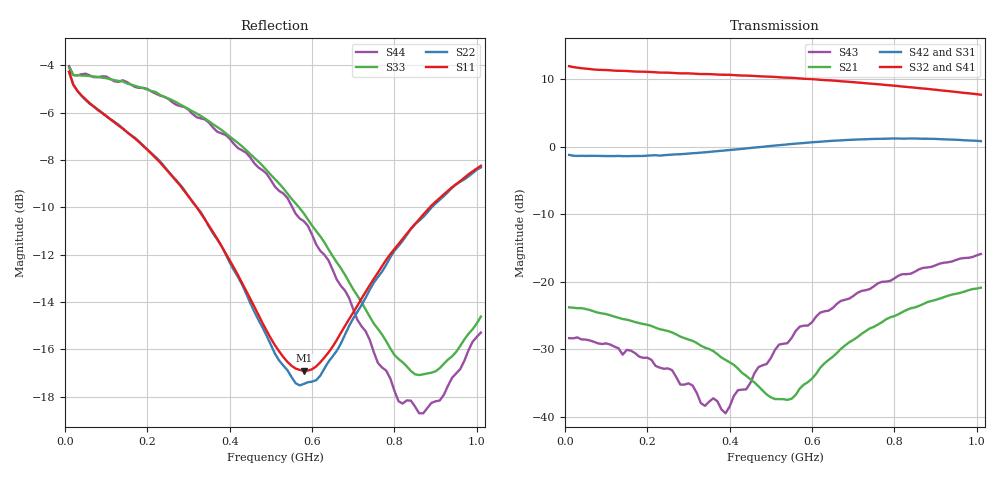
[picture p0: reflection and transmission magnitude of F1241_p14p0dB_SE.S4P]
! Integrated Device Technology
! Corporate Headquarters
! 6024 Silver Creek Valley Road
! San Jose, CA 95138  USA
! Phone:  1-408-284-8200
! Toll Free:  1-800-223-1366
! Webpage:  http://www.idt.com/
! Timing and RF Division
! 515 Groton Road, Suite 102
! Westford, MA 01886-6024
! Device:  F1241
! Description: Dual Intermediate Frequency Digital Variable Gain Amplifier
! Frequency:  10.0 -  500.00 MHz
! Package:  5x5 mm QFN Plastic Package: 32 pin
! Ports:  8 RF, 20 DC
!  Pin  1  = GA3  Pin 17  = RF OUT_B+
!  Pin  2  = GA4  Pin 18  = RF OUT_B-
!  Pin  3  = GA5  Pin 19  = STBY_B
!  Pin  4  = ISET_A  Pin 20  = Ground
!  Pin  5  = ISET_B  Pin 21  = Ground
!  Pin  6  = GB5  Pin 22  = STB_A
!  Pin  7  = GB4  Pin 23  = RF OUT_A-  = Port 4
!  Pin  8  = GB3  Pin 24  = RF OUT_A+  = Port 3
!  Pin  9  = GB2  Pin 25  = NO CONNECT
!  Pin 10  = GB1  Pin 26  = NO CONNECT
!  Pin 11  = RF IN_B+  Pin 27  = VCC
!  Pin 12  = RF IN_B-  Pin 28  = Ground
!  Pin 13  = Ground  Pin 29  = RF IN_A-  = Port 2
!  Pin 14  = VCC  Pin 30  = RF IN_A+  = Port 1
!  Pin 15  = NO CONNECT  Pin 31  = GA1
!  Pin 16  = NO CONNECT  Pin 32  = GA2
! State:  6
! Gain State:  14.0 dB
! Voltages:  Vcc = +5.00 Volts  Icc approximately 160.0 mA or 80 mA per channel.
! Data:  The device was measured on a custom evaluation board which has
!  individual transmission lines to the RF pins.  Data was collected
!  using a calibrated network analyzer.  The evaluation board was
!  de-embedded using a port reference technique.
!  The reference plane is the edge of the package pin.
!  Only Channel A was measured.
!  This data is in single-ended operation.  If your needs are balanced
!  or differential S-parameters then this file needs to be used a
!  linear simulator.
! Misc:  Lot Code  160028MY
!  Action Tracker AT004
! Date Measured:  2014-08-14
! Date:  2014-08-28  MJV
! Note:
!  Integrated Device Technology supplies this data as a sample of measured
!  data at the package pin for this product.  Your particular data for this
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# Hz S dB R 50
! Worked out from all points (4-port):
!   101 points, 10 MHz to 1.01 GHz, reference 50 ohm
!   strongest paths, dB at 10 MHz, 260 MHz, 510 MHz, 760 MHz, 1.01 GHz:
!     S32: 11.9, 10.9, 10.3, 9.2, 7.7
!     S41: 11.9, 10.9, 10.2, 9.1, 7.5
!     S42: -1.2, -1.2, 0.2, 1.2, 0.8
!     S31: -1.2, -1.3, -0.1, 0.9, 0.6
!     S21: -23.8, -27.5, -37.4, -26.4, -20.9
!     S43: -28.4, -33.1, -30.1, -20.2, -15.9
!   lowest |S11| = -16.9 dB at 580 MHz (marker M1), VSWR 1.33, Z = 39.5 - j7.36 ohm
!   |S11| at or under -10 dB: 319.9 MHz to 886 MHz (566.1 MHz wide, 93.9 % of centre)
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1e7  -4.28 -13.3  -23.83 7.1  -48.91 40.6  -21.33 8.6
     -23.81 7.1  -4.29 -13.2  -21.34 8.2  -48.87 41.7
     -1.24 2.3  11.92 -176.4  -4.11 -10.3  -28.44 21.7
     11.94 -176.3  -1.23 2.4  -28.37 20.8  -4.04 -10.5
5e7  -5.44 -14.5  -24.13 -10.0  -43.83 53.7  -21.61 -2.7
     -24.05 -9.8  -5.47 -14.1  -21.55 -2.7  -43.92 55.1
     -1.35 -3.5  11.56 172.0  -4.44 -6.0  -28.85 -4.6
     11.56 171.7  -1.37 -3.6  -28.57 -3.1  -4.36 -6.1
2.2e8  -7.92 -37.6  -26.86 -34.3  -33.02 56.4  -21.82 -9.4
       -26.82 -37.4  -7.87 -35.8  -21.82 -9.5  -33.07 56.0
       -1.38 -15.0  11.02 149.1  -5.13 -19.1  -31.50 -47.4
       10.99 148.5  -1.27 -14.8  -32.48 -44.9  -5.20 -18.3
3.9e8  -11.94 -67.8  -31.40 -62.0  -28.58 41.4  -21.34 -16.3
       -31.60 -69.0  -11.97 -65.1  -21.23 -16.1  -28.52 40.5
       -0.78 -25.1  10.65 127.9  -6.87 -33.9  -33.35 -120.9
       10.56 126.9  -0.56 -25.7  -39.50 -134.9  -6.94 -32.3
5.8e8  -16.89 -140.3  -39.98 166.7  -25.83 22.7  -20.75 -28.5
       -35.25 166.9  -17.45 -137.9  -20.52 -28.4  -25.72 20.9
       0.27 -42.0  10.06 103.6  -10.26 -55.3  -26.31 159.9
       9.92 102.7  0.54 -43.8  -26.52 133.9  -10.58 -51.4
8.1e8  -11.55 144.9  -25.92 96.6  -24.20 0.9  -20.74 -46.9
       -24.82 98.8  -11.63 144.2  -20.34 -46.9  -24.08 -2.0
       1.00 -69.7  8.96 74.9  -16.40 -106.7  -19.64 109.3
       8.76 74.1  1.20 -72.6  -19.11 96.8  -18.18 -107.2
1.01e9  -8.25 123.7  -21.60 72.0  -23.54 -15.6  -21.40 -61.8
        -20.89 71.7  -8.32 123.8  -20.87 -62.2  -23.42 -19.3
        0.62 -95.9  7.69 51.7  -14.61 -175.9  -16.43 77.7
        7.45 51.0  0.81 -99.3  -15.91 68.0  -15.29 176.4
